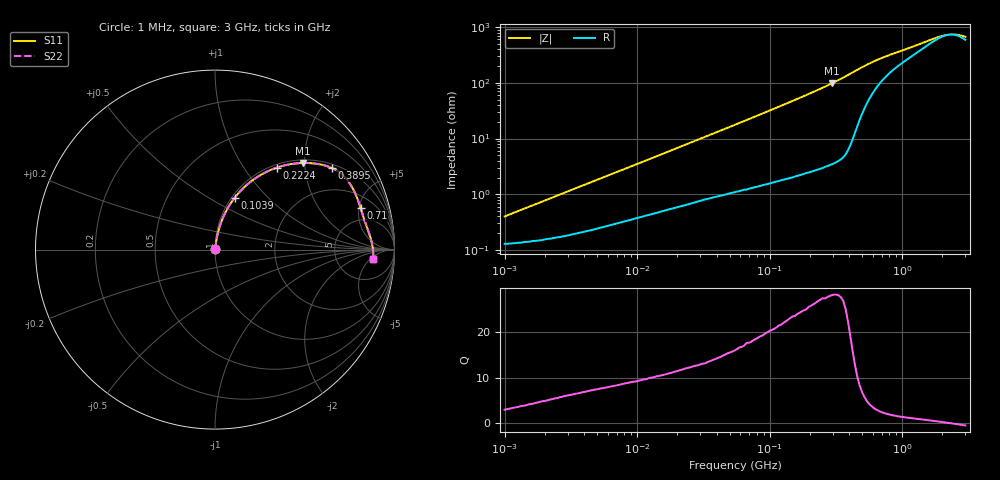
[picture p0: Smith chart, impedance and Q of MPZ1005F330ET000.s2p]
! S-Parameter Data Generated by TDK Corporation
! Copyright(C) 2025 TDK Corporation.
! All Rights Reserved.
! TDK P/N: MPZ1005F330ET000 (Chip Bead)
! Property: |Z|=33ohm at 100MHz
! Size(LxWxT): 1x0.5x0.5mm
! Model Type: s2p (Touchstone File Format Version 1.0)
! Frequency: DC=Yes Start=1MHz Stop=3000MHz 202points Log-sweep
! Model Generated on Feb. 6, 2025
! Terms and conditions regarding TDK Simulation Models:
! 1)This simulation model is being provided solely for informational
!  purposes. Please refer to the specifications of the products in
!  terms of detailed characteristics of such products.
! 2)In no event shall TDK Corporation of any of its subsidiaries be
!  liable for any loss or damage arising, directly or indirectly,
!  from any information contained in this simulation model, including,
!  but not limited to loss or damages arising from any inaccuracies,
!  omissions or errors in connection with such information.
! 3)Any and all copyrights on this simulation model are owned by
!  TDK Corporation.  Duplication or redistribution of this simulation
!  model without prior written permission from TDK Corporation
!  is prohibited.
! 4)This simulation model is subject to any modification or change
!  without any prior notice.
! 5)Neither TDK Corporation nor any of its subsidiaries shall make any
!  warranty, express or implied, including but not limited to the
!  correctness, implied warranties of merchantability and fitness for
!  a particular purpose with respect to this simulation models.
! 6)The use of this simulation model shall be deemed to have consented
!  to the terms and conditions hereof.
! Port Assignments:
!  1 ---@@@--- 2
! Applicable Conditions:
!  Temperature = 25 degC
!  DC Bias Current = 0 A
!  Small Signal Operation
# Hz S MA R 50
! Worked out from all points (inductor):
!   201 points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, 1 MHz to 3 GHz, reference 50 ohm
!   read as one part in series: L = 60.6 nH near 1.041 MHz
!   highest Q = 28.2 at 294.3 MHz (marker M1), where L = 52.7 nH
!   self-resonance near 2.28 GHz
!   S11 on the Smith chart (normalised r, x): 1 MHz: 1.00, +0.01; 103.9 MHz: 1.03, +0.66; 222.4 MHz: 1.05, +1.43; 389.5 MHz: 1.12, +2.76; 710 MHz: 3.23, +5.19; 3 GHz: 13, -6
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1000000  0.004007 71.0  0.9987 -0.2  0.9987 -0.2  0.004007 71.0
3900413  0.01443 80.8  0.9978 -0.8  0.9978 -0.8  0.01443 80.8
1.461624e7  0.04974 81.7  0.994 -2.8  0.994 -2.8  0.04974 81.7
3.00453e7  0.098 80.0  0.9877 -5.6  0.9877 -5.6  0.098 80.0
5.477226e7  0.1722 76.5  0.9744 -9.9  0.9744 -9.9  0.1722 76.5
7.852918e7  0.2404 73.0  0.9578 -13.9  0.9578 -13.9  0.2404 73.0
1.039275e8  0.3094 69.2  0.936 -18.0  0.936 -18.0  0.3094 69.2
1.49005e8  0.4214 62.7  0.8892 -24.9  0.8892 -24.9  0.4214 62.7
2.136344e8  0.5562 54.0  0.8101 -33.8  0.8101 -33.8  0.5562 54.0
2.223601e8  0.5722 53.0  0.7988 -34.9  0.7988 -34.9  0.5722 53.0
2.942768e8  0.6859 44.7  0.7038 -43.3  0.7038 -43.3  0.6859 44.7
3.453811e8  0.7499 39.4  0.6351 -48.5  0.6351 -48.5  0.7499 39.4
3.894533e8  0.7934 35.0  0.5746 -52.4  0.5746 -52.4  0.7934 35.0
4.391493e8  0.8238 30.4  0.5073 -55.2  0.5073 -55.2  0.8238 30.4
5.154121e8  0.8391 24.6  0.4215 -55.8  0.4215 -55.8  0.8391 24.6
7.099691e8  0.8437 15.9  0.2987 -50.8  0.2987 -50.8  0.8437 15.9
8.005644e8  0.8452 13.7  0.268 -48.2  0.268 -48.2  0.8452 13.7
2.01032e9  0.8768 1.6  0.126 -11.2  0.126 -11.2  0.8768 1.6
2.177892e9  0.879 0.6  0.1214 -4.3  0.1214 -4.3  0.879 0.6
2.455801e9  0.8815 -1.0  0.1195 7.1  0.1195 7.1  0.8815 -1.0
2.660507e9  0.8823 -2.0  0.1221 14.5  0.1221 14.5  0.8823 -2.0
3e9  0.8818 -3.5  0.1317 24.5  0.1317 24.5  0.8818 -3.5
